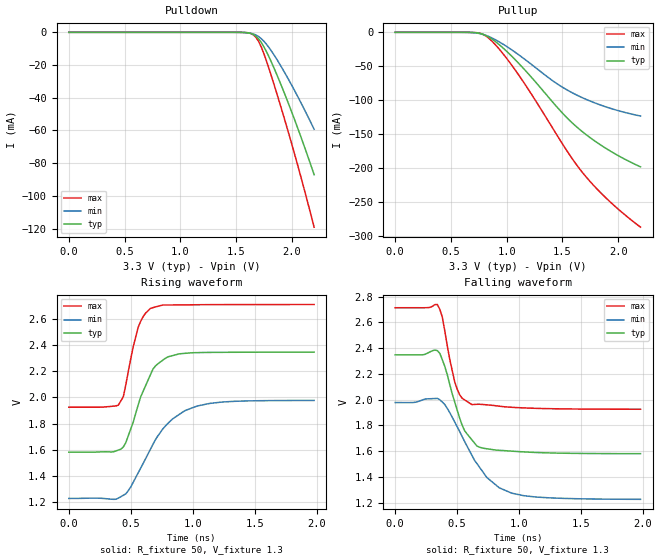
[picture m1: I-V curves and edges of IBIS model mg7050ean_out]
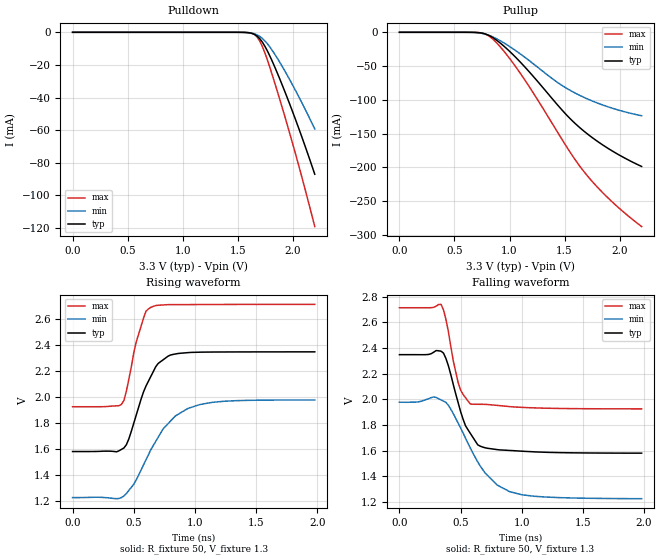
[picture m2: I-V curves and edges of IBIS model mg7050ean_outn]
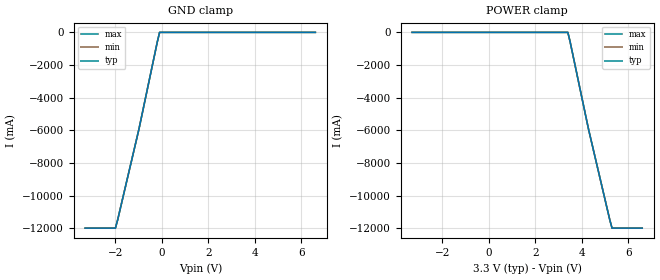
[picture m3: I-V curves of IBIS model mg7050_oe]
|   IBIS File mg7050ean_4out_33v.ibs
[IBIS Ver]   3.2
[Comment Char]   |_char
[File name]   mg7050ean_4out_33v.ibs
[File Rev]   1.0
[Date]   Aug 02, 2013
[Source]
|   Component MG7050EAN LV-PECL 4-OUTPUT 3.3V
[Component]   mg7050ean-pecl-4out
[Manufacturer]   Seiko Epson Corporation
[Package]
| variable   typ   min   max
R_pkg   0.27   NA   NA
L_pkg   1.66n   NA   NA
C_pkg   0.53p   NA   NA
[Pin]   signal_name   model_name   R_pin   L_pin   C_pin
1   vcc1   POWER   NA   NA   NA
2   out1p   mg7050ean_out   0.34   2.1nH   0.58pF
3   out1n   mg7050ean_outn  0.25   1.5nH   0.50pF
4   out2p   mg7050ean_out   0.22   1.3nH   0.44pF
5   out2n   mg7050ean_outn  0.25   1.7nH   0.59pF
6   fsel   mg7050_fsel   NA   NA   NA
7   oe   mg7050_oe   NA   NA   NA
8   out3n   mg7050ean_outn  0.25   1.7nH   0.62pF
9   out3p   mg7050ean_out   0.22   1.3nH   0.49pF
10   out4n   mg7050ean_outn  0.25   1.5nH   0.46pF
11   out4p   mg7050ean_out   0.34   2.1nH   0.57pF
12   vcc2   POWER   NA   NA   NA
13   vcc   POWER   NA   NA   NA
14   gnd   GND   NA   NA   NA
[Diff Pin] inv_pin vdiff   tdelay_typ
2   3   0   0
4   5   0   0
9   8   0   0
11   10   0   0
| Models and submodels in the file (4): mg7050ean_out (Output_ECL), mg7050ean_outn (Output_ECL), mg7050_oe (Input), mg7050_fsel (Input)
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[Model]   mg7050ean_out
Model_type Output_ECL
Enable Active-High
Polarity Non-Inverting
Vref=1.3
Vmeas=1.97
Rref=50
Cref=0
C_comp   0.121p   0.121p   0.121p
[Temperature Range] 25   90   -40
[Voltage Range]   3.3   2.97   3.63
[Pullup Reference]  3.3   2.97   3.63
[Pulldown Reference]3.3   2.97   3.63
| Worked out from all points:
|   falling waveform, R_fixture 50, V_fixture 1.3: 20-80 % time 160ps typ, 284ps min, 104ps max; typ from 2.35 V to 1.58 V
|   rising waveform, R_fixture 50, V_fixture 1.3: 20-80 % time 178ps typ, 294ps min, 110ps max; typ from 1.58 V to 2.35 V
[Pullup]
0V        395.4pA    479.2pA    434.8pA
700mV     -301.8uA   -539.1uA   -167.2uA
775mV     -2.235mA   -2.504mA   -2.213mA
825mV     -5.673mA   -5.207mA   -6.887mA
925mV     -17.17mA   -13.36mA   -23.27mA
1.075V    -40.2mA    -29.33mA   -55.33mA
1.225V    -66.98mA   -47.75mA   -92.09mA
1.45V     -110.1mA   -75.74mA   -151.5mA
1.575V    -131.7mA   -88.07mA   -183.5mA
1.675V    -146.1mA   -96.19mA   -205.9mA
1.9V      -172.3mA   -110.5mA   -245.9mA
2.2V      -198.5mA   -123.5mA   -287.4mA
[Pulldown]
0V        395.5pA    479pA      434.8pA
1.55V     -53.12uA   -69.03uA   -23.7uA
1.65V     -1.193mA   -887.1uA   -1.301mA
1.675V    -2.244mA   -1.53mA    -2.805mA
1.7V      -3.874mA   -2.491mA   -5.309mA
1.725V    -6.12mA    -3.815mA   -8.833mA
1.775V    -12.15mA   -7.496mA   -18.03mA
1.825V    -19.46mA   -12.22mA   -28.56mA
1.9V      -31.57mA   -20.43mA   -45.2mA
2V        -48.94mA   -32.51mA   -68.51mA
2.1V      -67.48mA   -45.51mA   -93.18mA
2.2V      -87.06mA   -59.29mA   -119.1mA
[Falling Waveform]
R_fixture=50
V_fixture=1.3
V_fixture_min=0.97
V_fixture_max=1.63
0s        2.348V     1.977V     2.713V
340ps     2.381V     2.01V      2.739V
380ps     2.31V      1.981V     2.642V
440ps     2.119V     1.9V       2.315V
500ps     1.92V      1.79V      2.082V
560ps     1.76V      1.675V     1.998V
620ps     1.687V     1.566V     1.961V
740ps     1.619V     1.395V     1.96V
940ps     1.6V       1.274V     1.941V
1.98ns    1.581V     1.226V     1.925V
[Rising Waveform]
R_fixture=50
V_fixture=1.3
V_fixture_min=0.97
V_fixture_max=1.63
0s        1.58V      1.225V     1.925V
400ps     1.597V     1.228V     1.941V
440ps     1.62V      1.249V     2.006V
520ps     1.811V     1.35V      2.39V
560ps     1.942V     1.422V     2.539V
660ps     2.177V     1.605V     2.684V
700ps     2.242V     1.678V     2.695V
820ps     2.317V     1.82V      2.71V
1.04ns    2.344V     1.935V     2.712V
1.98ns    2.348V     1.977V     2.713V
[Ramp]
R_load=50
dV/dt_r   4.606E-1/1.776E-10   4.513E-1/2.939E-10   4.729E-1/1.104E-10
dV/dt_f   4.606E-1/1.599E-10   4.513E-1/2.844E-10   4.729E-1/1.036E-10
|[End   mg7050ean_out
[Model]   mg7050ean_outn
Model_type Output_ECL
Enable Active-High
Polarity Inverting
Vref=1.3
Vmeas=1.97
Rref=50
Cref=0
C_comp   0.121p   0.121p   0.121p
[Temperature Range] 25   90   -40
[Voltage Range]   3.3   2.97   3.63
[Pullup Reference]  3.3   2.97   3.63
[Pulldown Reference]3.3   2.97   3.63
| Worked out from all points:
|   falling waveform, R_fixture 50, V_fixture 1.3: 20-80 % time 161ps typ, 280ps min, 102ps max; typ from 2.35 V to 1.58 V
|   rising waveform, R_fixture 50, V_fixture 1.3: 20-80 % time 180ps typ, 285ps min, 115ps max; typ from 1.58 V to 2.35 V
[Pullup]
0V        395.4pA    479.1pA    434.8pA
700mV     -301.8uA   -539.1uA   -167.2uA
775mV     -2.235mA   -2.504mA   -2.213mA
825mV     -5.673mA   -5.207mA   -6.887mA
925mV     -17.17mA   -13.36mA   -23.27mA
1.075V    -40.2mA    -29.33mA   -55.33mA
1.225V    -66.98mA   -47.75mA   -92.09mA
1.45V     -110mA     -75.73mA   -151.5mA
1.575V    -131.7mA   -88.07mA   -183.5mA
1.675V    -146.1mA   -96.19mA   -205.9mA
1.9V      -172.2mA   -110.5mA   -245.9mA
2.2V      -198.5mA   -123.5mA   -287.4mA
[Pulldown]
0V        395.5pA    479pA      434.8pA
1.55V     -53.12uA   -69.03uA   -23.7uA
1.65V     -1.193mA   -887.1uA   -1.301mA
1.675V    -2.244mA   -1.53mA    -2.805mA
1.7V      -3.874mA   -2.491mA   -5.309mA
1.725V    -6.12mA    -3.815mA   -8.833mA
1.775V    -12.15mA   -7.496mA   -18.03mA
1.825V    -19.46mA   -12.22mA   -28.56mA
1.9V      -31.57mA   -20.43mA   -45.2mA
2V        -48.94mA   -32.51mA   -68.5mA
2.1V      -67.48mA   -45.51mA   -93.18mA
2.2V      -87.06mA   -59.29mA   -119.1mA
[Falling Waveform]
R_fixture=50
V_fixture=1.3
V_fixture_min=0.97
V_fixture_max=1.63
0s        2.348V     1.977V     2.713V
340ps     2.375V     1.996V     2.739V
400ps     2.262V     1.954V     2.528V
480ps     1.974V     1.814V     2.131V
540ps     1.794V     1.698V     2.013V
580ps     1.734V     1.619V     1.963V
660ps     1.635V     1.482V     1.961V
800ps     1.608V     1.332V     1.953V
900ps     1.602V     1.281V     1.943V
1.98ns    1.581V     1.226V     1.925V
[Rising Waveform]
R_fixture=50
V_fixture=1.3
V_fixture_min=0.97
V_fixture_max=1.63
0s        1.58V      1.225V     1.925V
400ps     1.597V     1.225V     1.944V
440ps     1.633V     1.257V     2.046V
520ps     1.859V     1.361V     2.422V
600ps     2.084V     1.516V     2.66V
640ps     2.159V     1.594V     2.691V
700ps     2.259V     1.69V      2.707V
780ps     2.314V     1.794V     2.712V
1.04ns    2.345V     1.942V     2.712V
1.98ns    2.348V     1.977V     2.713V
[Ramp]
R_load=50
dV/dt_r   4.606E-1/1.796E-10   4.193E-1/2.860E-10   4.769E-1/1.153E-10
dV/dt_f   4.606E-1/1.609E-10   4.193E-1/2.758E-10   4.769E-1/9.191E-11
|[End   mg7050ean_outn
[Model]   mg7050_oe
Model_type Input
Vinh=2.31
Vinl=0.99
C_comp   3p   3p   3p
[Temperature Range] 25   90   -40
[Voltage Range]   3.3   2.97   3.63
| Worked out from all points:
|   GND clamp passes 1 mA (typ) near -0.10 V on its own axis
[GND Clamp]
-3.3V     -12A       -12A       -12A
-2V       -12A       -12A       -12A
-1.9V     -11.47A    -11.47A    -11.47A
-1V       -6A        -6A        -6A
-200mV    -592.5mA   -592.5mA   -592.5mA
-100mV    -33.15uA   -27.35uA   -40.33uA
6.6V      32.19uA    32.39uA    32.12uA
[POWER Clamp]
-3.3V     32.19uA    32.39uA    32.12uA
3.4V      -33.15uA   -27.35uA   -40.33uA
3.5V      -592.5mA   -592.5mA   -592.5mA
4.3V      -6A        -6A        -6A
5.2V      -11.47A    -11.47A    -11.47A
5.3V      -12A       -12A       -12A
6.6V      -12A       -12A       -12A
